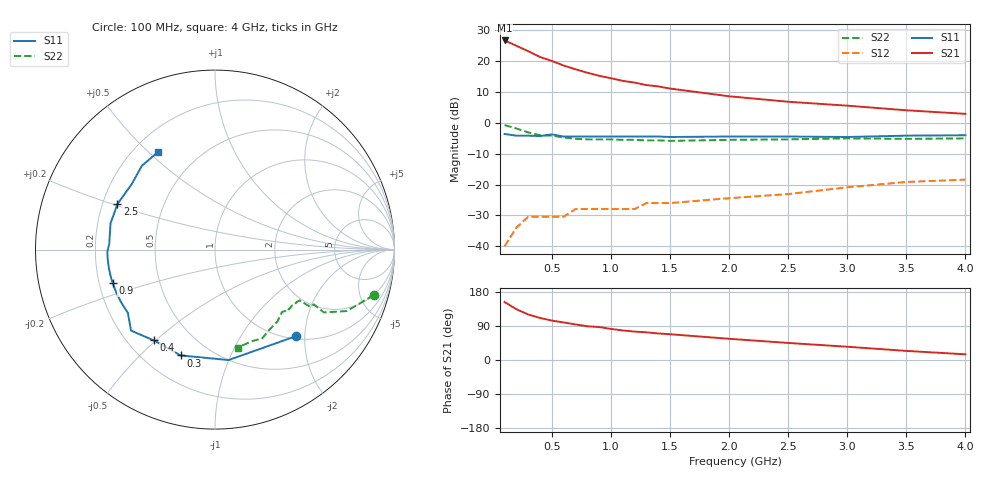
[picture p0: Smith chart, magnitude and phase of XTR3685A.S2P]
!  HXTR-3685 Typical S-Parameters
!  (Vce =10 V, Ic = 10 mA)
# ghz s ma r 50
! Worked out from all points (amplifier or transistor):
!   20 points, 100 MHz to 4 GHz, reference 50 ohm
!   highest |S21| = 26.7 dB at 100 MHz (marker M1)
!   |S21| within 3 dB of that: start of sweep to 271.8 MHz
!   unconditionally stable (mu >= 1): 1.084 GHz to 1.264 GHz; 1.393 GHz to 3.411 GHz; 3.883 GHz to end of sweep
!   at 400 MHz: K = 0.48, MSG = 25.9 dB, |S12| = -30.5 dB
!   at 1.1 GHz: K = 1.02, MAG = 19.9 dB, |S12| = -28.0 dB
!   at 4 GHz: K = 1.00, MAG = 10.3 dB, |S12| = -18.4 dB
!   S11 on the Smith chart (normalised r, x): 100 MHz: 1.05, -1.80; 300 MHz: 0.35, -0.67; 400 MHz: 0.31, -0.49; 900 MHz: 0.26, -0.15; 2.5 GHz: 0.26, +0.21; 4 GHz: 0.30, +0.54
0.1  0.66 -47.0  21.7 153.0  0.01 68.0  0.92 -16.0
0.2  0.62 -83.0  17.8 134.0  0.02 54.0  0.81 -25.0
0.3  0.62 -108.0  14.5 120.0  0.03 47.0  0.7 -30.0
0.4  0.61 -124.0  11.7 111.0  0.03 43.0  0.63 -29.0
0.5  0.65 -136.0  10.1 104.0  0.03 43.0  0.62 -31.0
0.6  0.6 -144.0  8.5 99.0  0.03 42.0  0.58 -31.0
0.7  0.6 -151.0  7.4 94.0  0.04 42.0  0.55 -31.0
0.8  0.6 -157.0  6.5 89.0  0.04 42.0  0.54 -33.0
0.9  0.6 -162.0  5.8 87.0  0.04 44.0  0.54 -33.0
1  0.6 -166.0  5.3 82.0  0.04 44.0  0.54 -35.0
1.1  0.6 -170.0  4.8 78.0  0.04 46.0  0.53 -36.0
1.2  0.6 -173.0  4.5 75.0  0.04 46.0  0.53 -39.0
1.3  0.6 -176.0  4.1 73.0  0.05 48.0  0.52 -39.0
1.4  0.6 -179.0  3.9 70.0  0.05 49.0  0.52 -41.0
1.5  0.59 177.0  3.6 68.0  0.05 50.0  0.51 -43.0
2  0.6 166.0  2.7 56.0  0.06 54.0  0.53 -49.0
2.5  0.6 155.0  2.2 45.0  0.07 57.0  0.54 -56.0
3  0.59 142.0  1.9 35.0  0.09 58.0  0.56 -62.0
3.5  0.62 131.0  1.6 24.0  0.11 58.0  0.55 -68.0
4  0.63 120.0  1.4 15.0  0.12 56.0  0.56 -77.0
